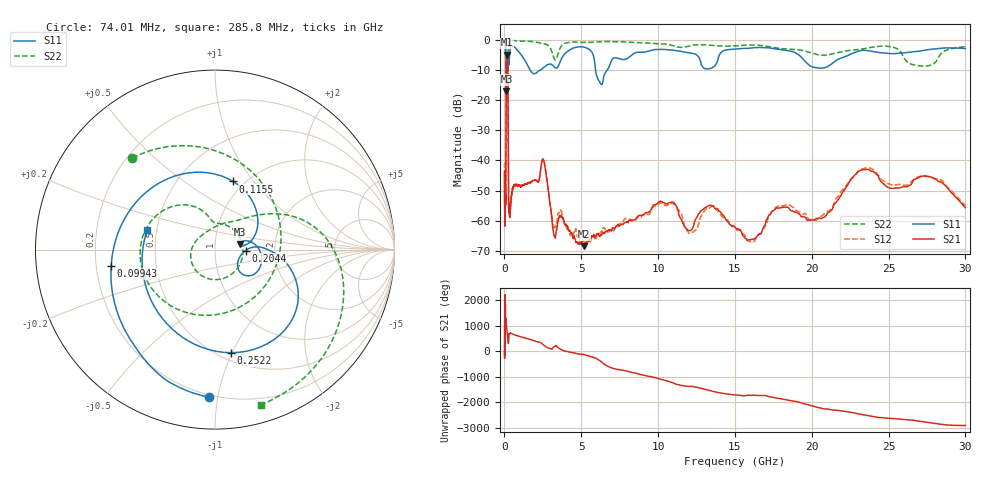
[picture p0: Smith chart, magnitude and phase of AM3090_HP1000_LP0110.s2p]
! Date/Time: Thu, Feb 28, 2019 2:02 PM
! Network Analyzer: Agilent Technologies E8364B Rev: A.07.50.67
! Sweep from 0.010 to 30.000 GHz, 1601 Points, Sweep Type: LOG
! Power Supply: 5.023 V, 0.002 A
# Hz S DB R 50
!freq MagS11 AngS11 MagS21 AngS21 MagS12 AngS12 MagS22 AngS22
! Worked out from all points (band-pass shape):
!   1601 points, 10 MHz to 30 GHz, reference 50 ohm
!   highest |S21| = -4.89 dB at 162.4 MHz (marker M1); lowest = -68.4 dB at 5.18 GHz (marker M2)
!   |S21| within 3 dB of the highest: 122.5 MHz to 213.5 MHz (91.02 MHz wide, 54.2 % of centre)
!   lowest |S11| = -17.0 dB at 131.6 MHz (marker M3), VSWR 1.33, Z = 65.9 + j3.86 ohm
!   |S11| at or under -10 dB: 119.3 MHz to 219.1 MHz (99.82 MHz wide, 59 % of centre); 1.668 GHz to 2.361 GHz (692.8 MHz wide, 34.4 % of centre); 5.925 GHz to 6.694 GHz (768.7 MHz wide, 12.2 % of centre)
!   |S22| runs from -19.3 to -0.2 dB; largest |S21 - S12| = 0.011
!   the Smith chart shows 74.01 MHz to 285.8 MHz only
!   S11 on the Smith chart (normalised r, x): 74.01 MHz: 0.18, -0.94; 99.43 MHz: 0.26, -0.07; 115.5 MHz: 0.89, +0.80; 204.4 MHz: 1.41, -0.02; 252.2 MHz: 0.57, -0.99; 285.8 MHz: 0.44, +0.12
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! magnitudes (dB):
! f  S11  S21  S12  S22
! 10 MHz  -0.2  -44.9  -40.6  -0.6
! 38.04 MHz  -0.5  -60.1  -60.2  -1.4
! 74.01 MHz  -1.7  -54.8  -52.1  -3.3
! 87.3 MHz  -2.9  -49.9  -51.6  -6.2
! 99.43 MHz  -4.6  -32.8  -32.7  -9.3
! 115.5 MHz  -8.1  -12.4  -12.4  -8.0
! 131.6 MHz  -17.0  -5.8  -5.8  -16.2
! 144.7 MHz  -12.8  -5.1  -5.1  -16.4
! 162.4 MHz  -11.4  -4.9  -4.8  -15.7
! 204.4 MHz  -15.4  -6.4  -6.4  -18.5
! 225.9 MHz  -8.2  -13.3  -13.3  -10.5
! 252.2 MHz  -4.7  -45.1  -45.2  -2.1
! 285.8 MHz  -8.1  -56.6  -54.4  -0.9
! 550.5 MHz  -2.0  -48.9  -49.2  -0.3
! 2.084 GHz  -10.9  -46.6  -46.6  -0.7
! 2.533 GHz  -9.2  -39.7  -39.6  -1.3
! 3.236 GHz  -8.9  -65.0  -62.5  -6.3
! 5.18 GHz  -2.4  -68.4  -67.3  -0.8
! 7.926 GHz  -6.3  -60.5  -59.2  -0.7
! 16.13 GHz  -2.7  -66.1  -66.7  -1.7
! 23.48 GHz  -3.5  -43.0  -42.5  -2.9
! 30 GHz  -2.8  -55.6  -54.9  -2.3
